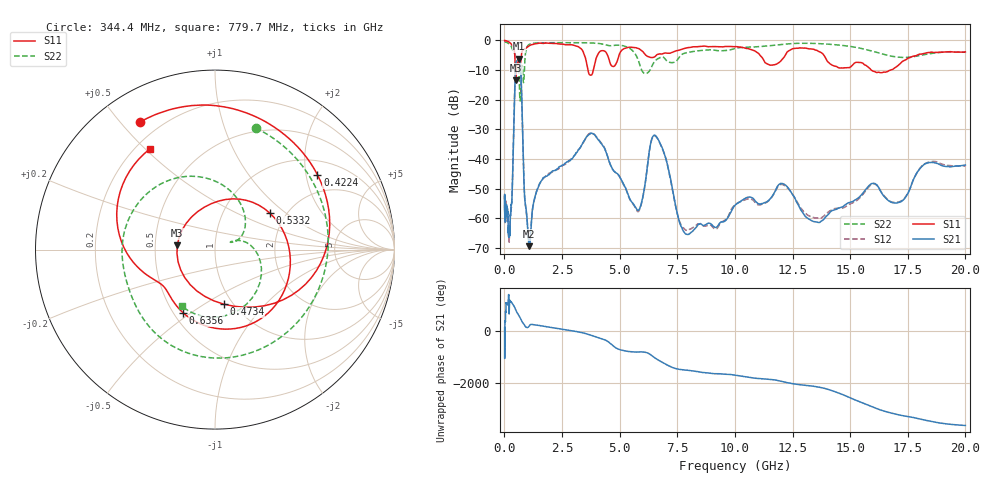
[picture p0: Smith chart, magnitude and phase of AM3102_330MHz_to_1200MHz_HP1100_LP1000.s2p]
! Date/Time: Tue, Sep 11, 2018 5:21 PM
! Network Analyzer: Agilent Technologies E8362B Rev: A.07.50.63
! Sweep from 0.010 to 20.000 GHz, 1601 Points, Sweep Type: LOG
! Power Supply: 4.949 V, 0.001 A
# Hz S DB R 50
!freq MagS11 AngS11 MagS21 AngS21 MagS12 AngS12 MagS22 AngS22
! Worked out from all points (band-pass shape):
!   1601 points, 10 MHz to 20 GHz, reference 50 ohm
!   highest |S21| = -6.17 dB at 626.6 MHz (marker M1); lowest = -69.5 dB at 1.082 GHz (marker M2)
!   |S21| within 3 dB of the highest: 484.6 MHz to 701.5 MHz (216.9 MHz wide, 36.6 % of centre)
!   lowest |S11| = -13.5 dB at 494.1 MHz (marker M3), VSWR 1.54, Z = 32.6 + j1.67 ohm
!   |S11| at or under -10 dB: 472.7 MHz to 521.2 MHz (48.57 MHz wide, 9.77 % of centre); 3.626 GHz to 3.86 GHz (234.1 MHz wide, 6.25 % of centre); 15.91 GHz to 16.77 GHz (856.5 MHz wide, 5.24 % of centre)
!   |S22| runs from -20.4 to -0.2 dB; largest |S21 - S12| = 0.0087
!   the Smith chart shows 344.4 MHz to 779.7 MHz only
!   S11 on the Smith chart (normalised r, x): 344.4 MHz: 0.13, +0.57; 422.4 MHz: 1.40, +2.33; 473.4 MHz: 0.91, -0.61; 533.2 MHz: 1.65, +0.78; 635.6 MHz: 0.56, -0.47; 779.7 MHz: 0.26, +0.52
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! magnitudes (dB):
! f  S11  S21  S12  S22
! 10 MHz  0.0  -52.6  -52.0  -0.2
! 35.55 MHz  -0.1  -59.3  -58.6  -0.4
! 126.4 MHz  -0.3  -57.8  -59.4  -0.8
! 210.1 MHz  -0.7  -64.0  -67.8  -1.2
! 344.4 MHz  -1.7  -49.7  -49.4  -2.9
! 422.4 MHz  -3.0  -23.7  -23.7  -4.3
! 447.2 MHz  -4.5  -16.6  -16.7  -4.4
! 473.4 MHz  -10.2  -10.8  -10.8  -5.0
! 494.1 MHz  -13.5  -8.2  -8.3  -5.5
! 533.2 MHz  -8.7  -7.0  -7.0  -5.8
! 626.6 MHz  -7.7  -6.2  -6.2  -10.4
! 635.6 MHz  -8.1  -6.2  -6.2  -11.7
! 779.7 MHz  -3.5  -26.9  -26.9  -8.7
! 873.8 MHz  -2.9  -52.3  -52.4  -9.3
! 1.082 GHz  -1.8  -69.5  -68.1  -1.3
! 1.59 GHz  -1.0  -47.5  -47.6  -0.8
! 3.811 GHz  -11.3  -31.4  -31.3  -0.9
! 5.652 GHz  -2.4  -55.8  -56.1  -4.3
! 6.549 GHz  -5.4  -32.1  -32.3  -6.8
! 7.958 GHz  -2.5  -65.5  -64.1  -4.1
! 13.61 GHz  -3.6  -61.4  -59.9  -1.1
! 20 GHz  -3.9  -42.1  -42.4  -4.0
